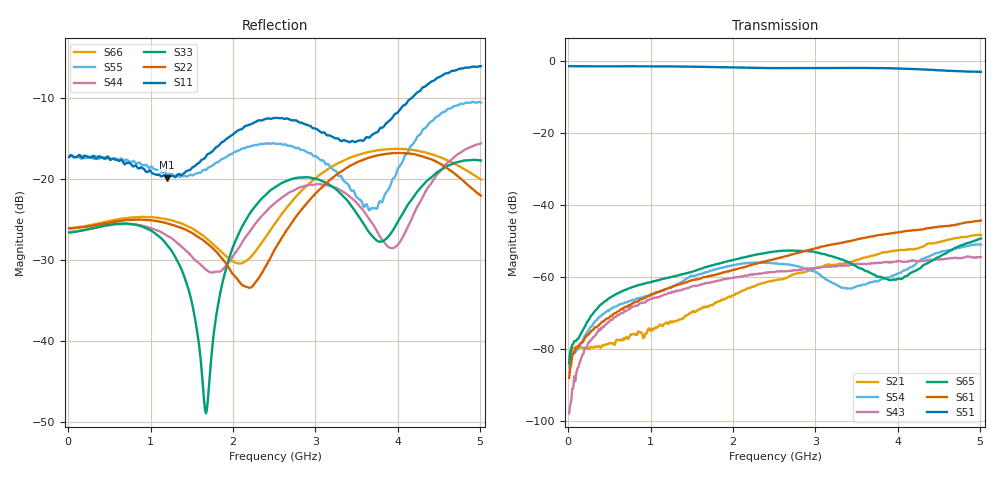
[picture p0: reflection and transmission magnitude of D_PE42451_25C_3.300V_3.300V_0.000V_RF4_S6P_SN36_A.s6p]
! Device ID: PE42451
! Serial: 36
! Insertion: A
! Temp: 25C
! VDD: 3.300
! Control_Hi: 100.000
! Control_Lo: 0.000
! Logic State: RF4
! Port 1: RFC
! Port 2: RF1
! Port 3: RF2
! Port 4: RF3
! Port 5: RF4
! Port 6: RF5
! V1 = 0.00
! V2 = 0.00
! V3 = 3.30
! V4 = 0.00
! IDD: 1.592240e-05
#  Hz  S  RI  R  50
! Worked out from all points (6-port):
!   401 points, 10 MHz to 5.01 GHz, reference 50 ohm
!   strongest paths, dB at 10 MHz, 1.26 GHz, 2.51 GHz, 3.76 GHz, 5.01 GHz:
!     S51: -1.4, -1.5, -2.0, -2.0, -3.0
!     S61: -87.9, -62.7, -54.9, -48.3, -44.2
!     S65: -83.9, -59.9, -52.8, -59.9, -49.2
!     S43: -97.7, -63.9, -58.5, -56.1, -54.4
!     S54: -85.0, -62.6, -56.1, -61.2, -50.9
!     S21: -83.5, -72.6, -60.9, -53.6, -48.3
!   lowest |S11| = -19.9 dB at 1.198 GHz (marker M1), VSWR 1.23, Z = 55.4 - j9.28 ohm
!   |S11| at or under -10 dB: start of sweep to 4.175 GHz
